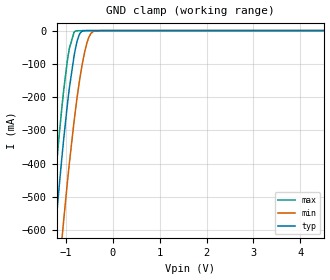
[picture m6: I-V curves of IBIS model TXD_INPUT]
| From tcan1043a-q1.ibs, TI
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|   TXD_INPUT Model
[Model]   TXD_INPUT
Model_type   Input
Vinl = 0.99
Vinh = 2.31
|   typ   min   max
C_comp   1.526pF   1.323pF   1.651pF
|  Where Nom  PVT is Nominal Process,   3.3V,  27C
|   Fast PVT is Strong Process,   5.5V, -55C
|   Slow PVT is Weak Process,   2.8V, 150C
[Model spec]
|subparameter
Vinl   0.990   0.840   1.650
Vinh   2.310   1.960   3.850
[Voltage Range]   3.3   2.8   5.5
|Junction Temperature
[Temperature Range]   27   150   -55
[Power Clamp Reference]   3.3   2.8   5.5
[GND Clamp Reference]   0   0   0
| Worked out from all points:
|   GND clamp passes 1 mA (typ) near -0.63 V on its own axis
[GND Clamp]
|   Voltage   I(typ)   I(min)   I(max)
-3.3V     -4.563A    -4.77A     -4.442A
-1.327V   -775mA     -1.025A    -620.1mA
-1.248V   -639mA     -890mA     -482.9mA
-1.182V   -530mA     -780.6mA   -374.1mA
-1.087V   -383.2mA   -630.1mA   -232.4mA
-1.045V   -322.7mA   -566.2mA   -176.6mA
-927.2mV  -173.8mA   -399.8mA   -54.21mA
-797.6mV  -54.91mA   -240.4mA   -1.67mA
-710.6mV  -11.23mA   -151.5mA   -268.6uA
-602.7mV  -454.5uA   -66.49mA   -103.3uA
-408.7mV  -17.07uA   -2.186mA   -90.68uA
6.6V      0A         0A         0A
[POWER Clamp]
|   Voltage   I(typ)   I(min)   I(max)
-3.3V     0A         0A         0A
0V        0A         0A         0A
6.6V      0A         0A         0A
